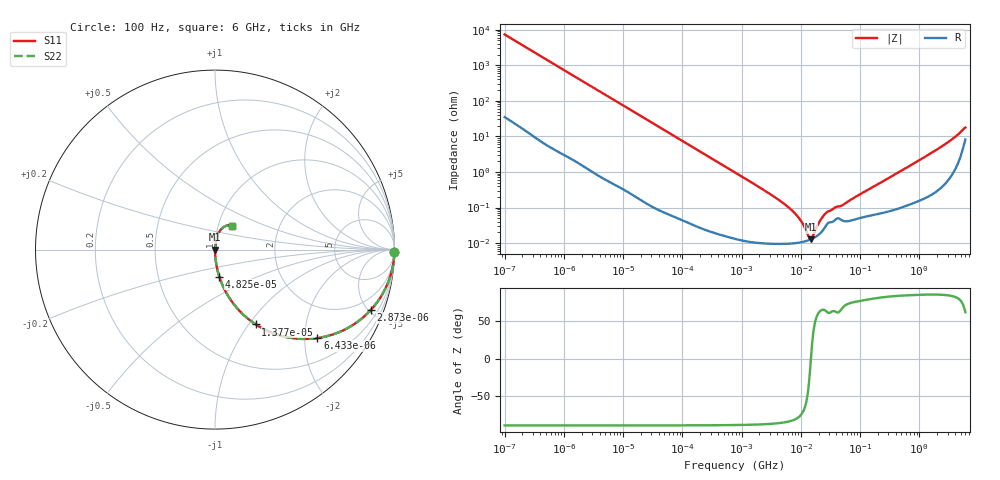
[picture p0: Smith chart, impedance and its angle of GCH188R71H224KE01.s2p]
!Murata Part Number: GCH188R71H224KE01
!These Parameters are Measured in Series Mode Connection
!Data Generated on Jun 19, 2026
!  o--ll--o
!Port1  Port2
!  o------o
!Operation Temp=25[degC], DC Bias Voltage=0[V]
!Freq. Start=100[Hz] Stop=6[GHz] 401[Steps]
# Hz S RI R 50
!Freq.(Hz) S11(Real) S11(Imag) S21(Real) S21(Imag) S12(Real) S12(Imag) S22(Real) S22(Imag)
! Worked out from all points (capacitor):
!   401 points, 100 Hz to 6 GHz, reference 50 ohm
!   read as one part in series: C = 216 nF near 109 Hz
!   lowest |Z| = 12.8 mohm at 14.88 MHz (marker M1)
!   series resonance near 14.81 MHz, so ESL is about 530 pH
!   S11 on the Smith chart (normalised r, x): 100 Hz: open; 2.873 kHz: 1.02, -5.16; 6.433 kHz: 1.01, -2.31; 13.77 kHz: 1.00, -1.08; 48.25 kHz: 1.00, -0.31; 6 GHz: 1.16, +0.31
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100  0.9998 -0.0136  0.00025 0.0136  0.00025 0.0136  0.9998 -0.0136
600  0.9931 -0.0806  0.00686 0.0806  0.00686 0.0806  0.9931 -0.0806
2008  0.9306 -0.2521  0.0694 0.2521  0.0694 0.2521  0.9306 -0.2521
2873  0.8684 -0.3361  0.1316 0.3361  0.1316 0.3361  0.8684 -0.3361
6433  0.5711 -0.4928  0.4289 0.4928  0.4289 0.4928  0.5711 -0.4928
13772  0.2271 -0.4168  0.7729 0.4168  0.7729 0.4168  0.2271 -0.4168
22537  0.0996 -0.2973  0.9004 0.2973  0.9004 0.2973  0.0996 -0.2973
40335  0.0339 -0.1786  0.9661 0.1786  0.9661 0.1786  0.0339 -0.1786
48246  0.0241 -0.1509  0.9759 0.1509  0.9759 0.1509  0.0241 -0.1509
147774  0.00289 -0.0505  0.9971 0.0505  0.9971 0.0505  0.00289 -0.0505
774597  0.000225 -0.0097  0.9998 0.0097  0.9998 0.0097  0.000225 -0.0097
3103719  0.000101 -0.00233  0.9999 0.00233  0.9999 0.00233  0.000101 -0.00233
6353432  9.72e-05 -0.000974  0.9999 0.000974  0.9999 0.000974  9.72e-05 -0.000974
9506416  0.000104 -0.00047  0.9999 0.00047  0.9999 0.00047  0.000104 -0.00047
1.360128e7  0.000121 -8.79e-05  0.9999 8.79e-05  0.9999 8.79e-05  0.000121 -8.79e-05
1.487547e7  0.000128 4.7e-06  0.9999 -4.7e-06  0.9999 -4.7e-06  0.000128 4.7e-06
1.555665e7  0.000132 5.11e-05  0.9999 -5.11e-05  0.9999 -5.11e-05  0.000132 5.11e-05
2.128304e7  0.000188 0.000389  0.9998 -0.000389  0.9998 -0.000389  0.000188 0.000389
2.784235e7  0.000344 0.000663  0.9997 -0.000663  0.9997 -0.000663  0.000344 0.000663
3.124326e8  0.00083 0.00687  0.9992 -0.00687  0.9992 -0.00687  0.00083 0.00687
2.240541e9  0.0057 0.0481  0.9943 -0.0481  0.9943 -0.0481  0.0057 0.0481
6e9  0.0948 0.1316  0.9052 -0.1316  0.9052 -0.1316  0.0948 0.1316
